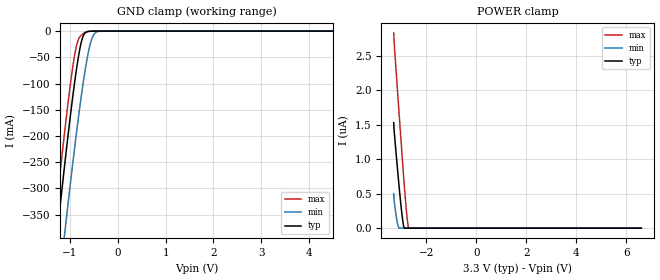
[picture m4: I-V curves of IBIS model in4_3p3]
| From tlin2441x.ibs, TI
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|   in4_3p3 Model
[Model]   in4_3p3
Model_type   Input
Vinl = 0.66
Vinh = 2.64
|   typ   min   max
C_comp   4.302pF   4.223pF   4.504pF
|  Where Nom  PVT is Nominal Process, 3.3V,   27C
|   Fast PVT is Strong Process,  3.6,   -40C
|   Slow PVT is Weak Process,   3.0V,   150C
[Model spec]
|subparameter
Vinl   0.66   0.6   0.72
Vinh   2.64   2.4   2.88
[Voltage Range]   3.3   3   3.6
|Junction Temperature
[Temperature Range]   27   150   -40
[Power Clamp Reference]   3.3   3   3.6
[GND Clamp Reference]   0   0   0
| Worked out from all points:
|   GND clamp passes 1 mA (typ) near -0.63 V on its own axis
[GND Clamp]
|   Voltage   I(typ)   I(min)   I(max)
-3.3V     -2.208A    -2.294A    -2.167A
-1.33V    -437mA     -566.9mA   -373.8mA
-1.231V   -353.1mA   -484mA     -289.3mA
-1.102V   -247.3mA   -378.4mA   -183.9mA
-983.4mV  -154.8mA   -283.9mA   -95.2mA
-884.4mV  -85.28mA   -208.5mA   -36.2mA
-775.5mV  -25.56mA   -131.6mA   -8.893mA
-676.5mV  -2.938mA   -70.74mA   -2.425mA
-597.3mV  -421uA     -32.6mA    -493.6uA
-537.9mV  -105uA     -13.42mA   -119.2uA
-399.3mV  -15.24uA   -536.4uA   -16.65uA
6.6V      0A         0A         0A
[POWER Clamp]
|   Voltage   I(typ)   I(min)   I(max)
-3.3V     1.529uA    500.7nA    2.833uA
-3.29V    1.444uA    425.7nA    2.739uA
-3.231V   1.194uA    252.3nA    2.424uA
-3.132V   789.5nA    44.01nA    1.906uA
-3.092V   633.5nA    2.114nA    1.701uA
-3.003V   305.8nA    0A         1.244uA
-2.944V   122.8nA    0A         947.3nA
-2.884V   2.864nA    0A         659.4nA
-2.795V   0A         0A         263.5nA
-2.746V   0A         0A         89.32nA
-2.706V   0A         0A         3.64nA
6.6V      0A         0A         0A
